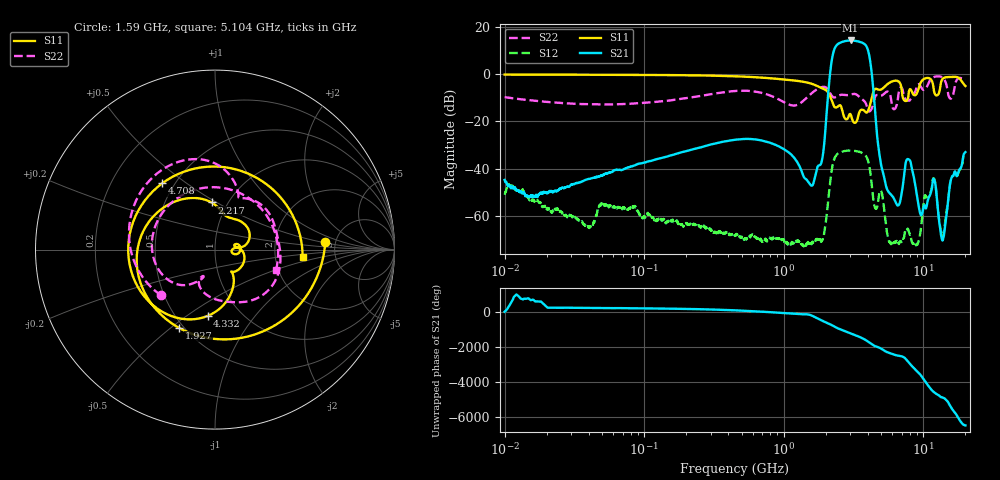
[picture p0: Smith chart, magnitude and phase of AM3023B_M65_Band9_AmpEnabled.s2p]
!Agilent Technologies,E8364B,MY43040894,A.07.50.67
!Agilent E8364B: A.07.50.67
!Date: Tuesday, October 27, 2020 10:54:31
!Correction: S11(Full 2 Port(1,2))
!S21(Full 2 Port(1,2))
!S12(Full 2 Port(1,2))
!S22(Full 2 Port(1,2))
!S2P File: Measurements: S11, S21, S12, S22:Log Frequency Sweep
# Hz S  dB  R 50
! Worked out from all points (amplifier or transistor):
!   3201 points, 10 MHz to 20 GHz, reference 50 ohm
!   highest |S21| = 14.1 dB at 3.012 GHz (marker M1)
!   |S21| within 3 dB of that: 2.332 GHz to 3.949 GHz (1.618 GHz wide, 51.5 % of centre)
!   unconditionally stable (mu >= 1): start of sweep to end of sweep
!   at 35.47 MHz: K = 8899.50, MAG = -34.3 dB, |S12| = -62.1 dB
!   at 447.2 MHz: K = 5445.22, MAG = -20.0 dB, |S12| = -68.5 dB
!   at 20 GHz: K = 331.52, MAG = -28.0 dB, |S12| = -33.5 dB
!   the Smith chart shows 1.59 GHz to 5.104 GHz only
!   S11 on the Smith chart (normalised r, x): 1.59 GHz: 4.12, +0.59; 1.927 GHz: 0.47, -0.54; 2.217 GHz: 0.84, +0.47; 4.332 GHz: 0.71, -0.61; 4.708 GHz: 0.43, +0.41; 5.104 GHz: 2.88, -0.32
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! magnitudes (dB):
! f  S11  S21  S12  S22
! 10 MHz  -0.3  -44.8  -51.1  -9.8
! 35.55 MHz  -0.3  -45.6  -62.3  -12.7
! 126.1 MHz  -0.5  -35.8  -61.8  -11.7
! 447.2 MHz  -1.0  -27.8  -68.5  -7.2
! 986.3 MHz  -2.3  -31.6  -69.9  -11.7
! 1.59 GHz  -4.2  -47.2  -71.3  -8.1
! 1.927 GHz  -6.4  -32.1  -68.5  -5.5
! 2.217 GHz  -11.6  6.5  -39.8  -9.4
! 3.012 GHz  -17.1  14.1  -32.4  -8.7
! 3.902 GHz  -16.4  11.7  -35.0  -13.0
! 4.332 GHz  -8.6  -3.6  -50.8  -13.6
! 4.708 GHz  -6.5  -28.5  -55.1  -9.0
! 5.104 GHz  -6.2  -41.0  -52.2  -8.9
! 5.639 GHz  -4.0  -49.9  -70.4  -7.7
! 6.675 GHz  -3.3  -55.4  -71.9  -7.4
! 7.789 GHz  -9.8  -36.0  -66.0  -11.3
! 8.94 GHz  -8.4  -50.5  -71.9  -5.5
! 9.692 GHz  -3.1  -59.7  -63.3  -5.9
! 11.86 GHz  -6.6  -44.4  -44.1  -1.4
! 13.74 GHz  -2.1  -70.2  -69.1  -1.6
! 15.85 GHz  -1.3  -44.2  -44.1  -10.3
! 20 GHz  -5.1  -33.1  -33.5  -2.6
